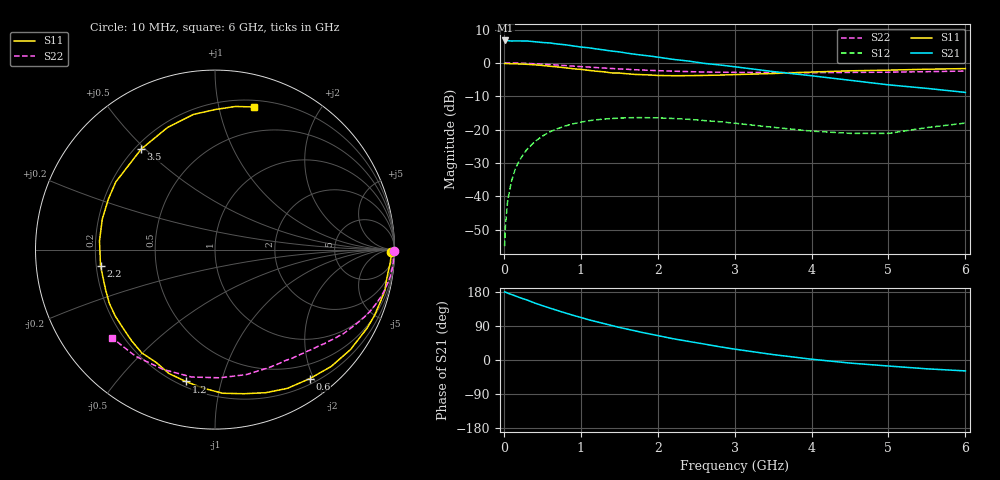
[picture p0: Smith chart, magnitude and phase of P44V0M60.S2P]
! SIEMENS Small Signal Semiconductors
! BFP182
! Si NPN RF Bipolar Junction Transistor in SOT143
! VCE = 4 V  IC = 0.6 mA
! Common Emitter S-Parameters:  March  1996
# GHz  S  MA  R  50
!  f  S11  S21  S12  S22
! GHz  MAG  ANG  MAG  ANG  MAG  ANG  MAG  ANG
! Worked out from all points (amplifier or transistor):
!   36 points, 10 MHz to 6 GHz, reference 50 ohm
!   highest |S21| = 6.7 dB at 20 MHz (marker M1)
!   |S21| within 3 dB of that: start of sweep to 1.348 GHz
!   unconditionally stable (mu >= 1): 2.894 GHz to end of sweep
!   at 250 MHz: K = 0.09, MSG = 17.1 dB, |S12| = -27.5 dB
!   at 1.4 GHz: K = 0.50, MSG = 10.1 dB, |S12| = -16.6 dB
!   at 6 GHz: K = 1.16, MAG = 2.2 dB, |S12| = -18.0 dB
!   S11 on the Smith chart (normalised r, x): 10 MHz: 66, -44; 600 MHz: 0.28, -1.94; 1.2 GHz: 0.23, -0.78; 2.2 GHz: 0.22, -0.07; 3.5 GHz: 0.22, +0.49; 6 GHz: 0.26, +1.28
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0.01  0.9794 -0.8  2.139 179.6  0.0018 78.8  0.9987 -0.3
0.02  0.9828 -1.9  2.173 179.2  0.0035 86.9  0.9999 -0.7
0.05  0.9784 -4.6  2.157 176.5  0.0087 85.5  0.9979 -1.6
0.1  0.9706 -9.1  2.133 172.8  0.017 83.8  0.9962 -3.3
0.15  0.9734 -13.9  2.139 169.1  0.0261 80.5  0.9953 -5.1
0.3  0.9538 -27.3  2.134 158.5  0.0507 71.9  0.9833 -10.0
0.4  0.9382 -36.4  2.08 150.5  0.0659 66.4  0.9734 -13.1
0.6  0.892 -53.7  1.993 136.9  0.0933 55.2  0.9449 -18.9
0.8  0.8458 -70.5  1.872 124.1  0.1139 45.2  0.9132 -24.3
1.1  0.7752 -94.8  1.689 106.4  0.1361 32.3  0.8678 -31.1
1.2  0.7526 -102.5  1.625 101.3  0.1407 27.9  0.854 -33.4
1.4  0.7092 -117.4  1.508 91.1  0.1472 20.9  0.827 -37.1
1.6  0.6887 -132.3  1.403 81.6  0.1509 14.8  0.8045 -40.6
1.9  0.6605 -153.0  1.268 68.6  0.1512 6.5  0.7753 -45.8
2.2  0.6441 -172.0  1.132 56.2  0.1472 -0.2  0.753 -50.9
2.8  0.6574 154.7  0.935 35.1  0.1321 -10.1  0.7272 -61.6
3.5  0.6947 126.3  0.743 14.3  0.1087 -14.4  0.7179 -76.0
4  0.7302 111.2  0.643 2.1  0.0952 -10.2  0.7147 -87.8
4.5  0.7626 99.1  0.55 -8.1  0.0882 -3.4  0.7217 -100.4
5  0.7804 89.9  0.47 -15.9  0.088 9.5  0.7273 -113.3
5.5  0.8055 81.9  0.416 -23.3  0.1077 15.0  0.7411 -126.7
6  0.8234 74.8  0.362 -28.8  0.1257 15.8  0.7555 -139.5
